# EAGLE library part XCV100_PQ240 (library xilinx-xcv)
xcv100_pq240_1532 edit this description Auto generated by make-symbol-device-package-bsdl.ulp Rev. 26 Source: xcv100_pq240_1532.bsd
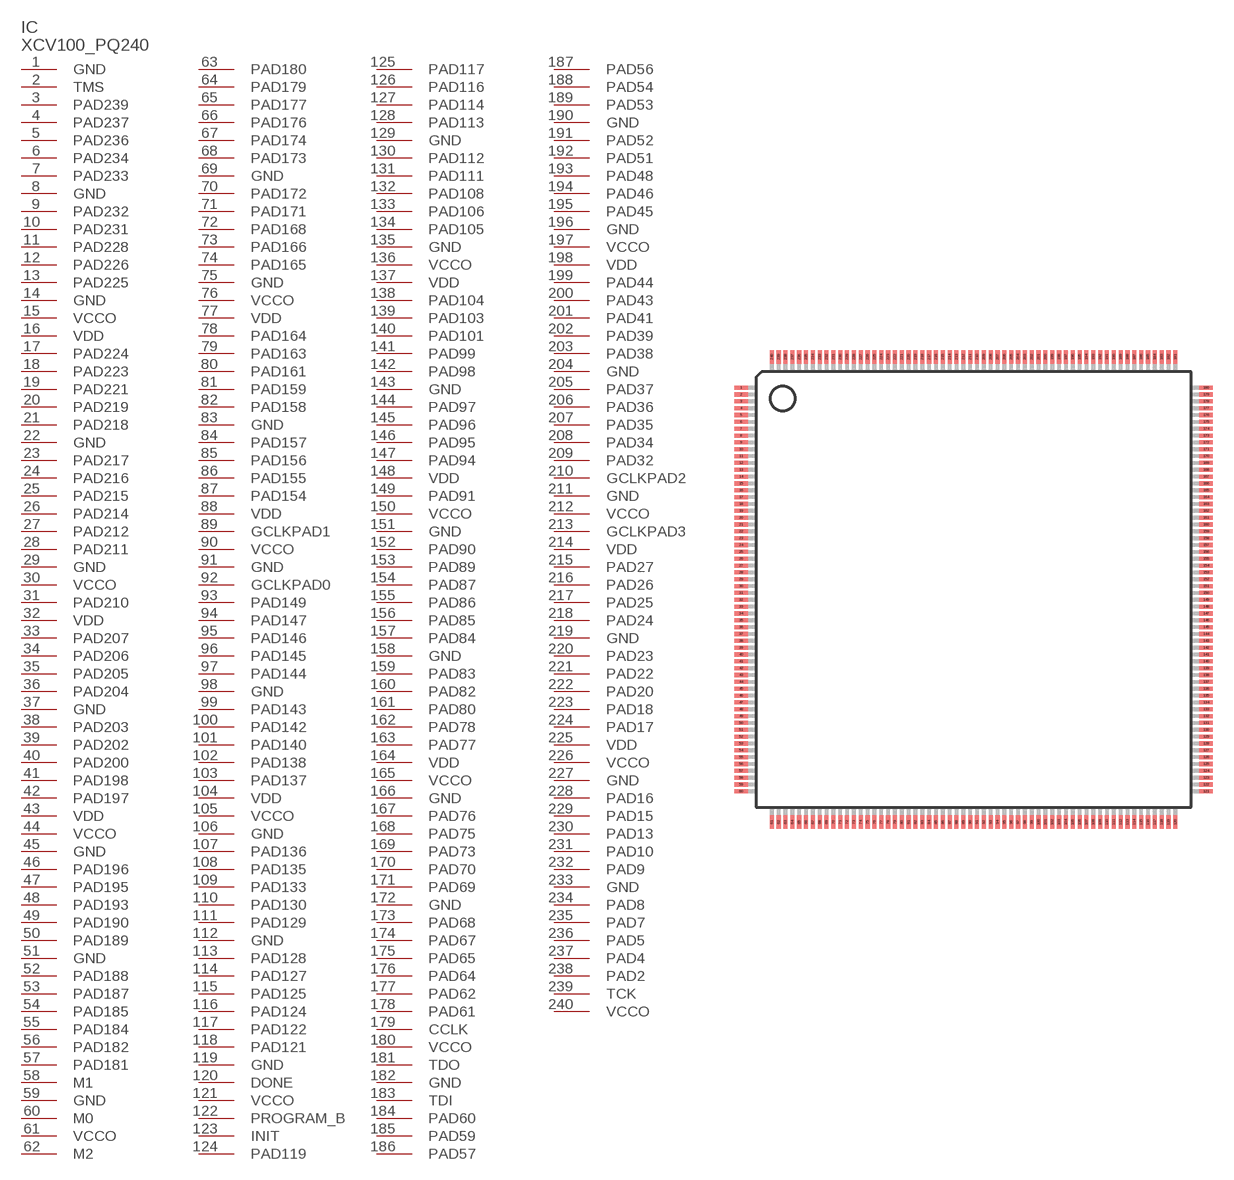
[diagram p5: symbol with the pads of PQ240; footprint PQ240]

Designator prefix IC

## XCV100_PQ240 (OC_FARNELL: unknown; OC_NEWARK: unknown)  [PQ240]
1  GND  pwr
2  TMS  in
3  PAD239
4  PAD237
5  PAD236
6  PAD234
7  PAD233
8  GND  pwr
9  PAD232
10  PAD231
11  PAD228
12  PAD226
13  PAD225
14  GND  pwr
15  VCCO  pwr
16  VDD  pwr
17  PAD224
18  PAD223
19  PAD221
20  PAD219
21  PAD218
22  GND  pwr
23  PAD217
24  PAD216
25  PAD215
26  PAD214
27  PAD212
28  PAD211
29  GND  pwr
30  VCCO  pwr
31  PAD210
32  VDD  pwr
33  PAD207
34  PAD206
35  PAD205
36  PAD204
37  GND  pwr
38  PAD203
39  PAD202
40  PAD200
41  PAD198
42  PAD197
43  VDD  pwr
44  VCCO  pwr
45  GND  pwr
46  PAD196
47  PAD195
48  PAD193
49  PAD190
50  PAD189
51  GND  pwr
52  PAD188
53  PAD187
54  PAD185
55  PAD184
56  PAD182
57  PAD181
58  M1  in
59  GND  pwr
60  M0  in
61  VCCO  pwr
62  M2  in
63  PAD180
64  PAD179
65  PAD177
66  PAD176
67  PAD174
68  PAD173
69  GND  pwr
70  PAD172
71  PAD171
72  PAD168
73  PAD166
74  PAD165
75  GND  pwr
76  VCCO  pwr
77  VDD  pwr
78  PAD164
79  PAD163
80  PAD161
81  PAD159
82  PAD158
83  GND  pwr
84  PAD157
85  PAD156
86  PAD155
87  PAD154
88  VDD  pwr
89  GCLKPAD1  in
90  VCCO  pwr
91  GND  pwr
92  GCLKPAD0  in
93  PAD149
94  PAD147
95  PAD146
96  PAD145
97  PAD144
98  GND  pwr
99  PAD143
100  PAD142
101  PAD140
102  PAD138
103  PAD137
104  VDD  pwr
105  VCCO  pwr
106  GND  pwr
107  PAD136
108  PAD135
109  PAD133
110  PAD130
111  PAD129
112  GND  pwr
113  PAD128
114  PAD127
115  PAD125
116  PAD124
117  PAD122
118  PAD121
119  GND  pwr
120  DONE
121  VCCO  pwr
122  PROGRAM_B  in
123  INIT
124  PAD119
125  PAD117
126  PAD116
127  PAD114
128  PAD113
129  GND  pwr
130  PAD112
131  PAD111
132  PAD108
133  PAD106
134  PAD105
135  GND  pwr
136  VCCO  pwr
137  VDD  pwr
138  PAD104
139  PAD103
140  PAD101
141  PAD99
142  PAD98
143  GND  pwr
144  PAD97
145  PAD96
146  PAD95
147  PAD94
148  VDD  pwr
149  PAD91
150  VCCO  pwr
151  GND  pwr
152  PAD90
153  PAD89
154  PAD87
155  PAD86
156  PAD85
157  PAD84
158  GND  pwr
159  PAD83
160  PAD82
161  PAD80
162  PAD78
163  PAD77
164  VDD  pwr
165  VCCO  pwr
166  GND  pwr
167  PAD76
168  PAD75
169  PAD73
170  PAD70
171  PAD69
172  GND  pwr
173  PAD68
174  PAD67
175  PAD65
176  PAD64
177  PAD62
178  PAD61
179  CCLK
180  VCCO  pwr
181  TDO  out
182  GND  pwr
183  TDI  in
184  PAD60
185  PAD59
186  PAD57
187  PAD56
188  PAD54
189  PAD53
190  GND  pwr
191  PAD52
192  PAD51
193  PAD48
194  PAD46
195  PAD45
196  GND  pwr
197  VCCO  pwr
198  VDD  pwr
199  PAD44
200  PAD43
201  PAD41
202  PAD39
203  PAD38
204  GND  pwr
205  PAD37
206  PAD36
207  PAD35
208  PAD34
209  PAD32
210  GCLKPAD2  in
211  GND  pwr
212  VCCO  pwr
213  GCLKPAD3  in
214  VDD  pwr
215  PAD27
216  PAD26
217  PAD25
218  PAD24
219  GND  pwr
220  PAD23
221  PAD22
222  PAD20
223  PAD18
224  PAD17
225  VDD  pwr
226  VCCO  pwr
227  GND  pwr
228  PAD16
229  PAD15
230  PAD13
231  PAD10
232  PAD9
233  GND  pwr
234  PAD8
235  PAD7
236  PAD5
237  PAD4
238  PAD2
239  TCK  in
240  VCCO  pwr

## Footprint PQ240 (pad centres in mm)
PQ240 Auto generated by make-symbol-device-package-bsdl.ulp Rev. 26
smd 1 x 0.3: 1 -17,14.75; 2 -17,14.25; 3 -17,13.75; 4 -17,13.25; 5 -17,12.75; 6 -17,12.25; 7 -17,11.75; 8 -17,11.25; 9 -17,10.75; 10 -17,10.25; 11 -17,9.75; 12 -17,9.25; 13 -17,8.75; 14 -17,8.25; 15 -17,7.75; 16 -17,7.25; 17 -17,6.75; 18 -17,6.25; 19 -17,5.75; 20 -17,5.25; 21 -17,4.75; 22 -17,4.25; 23 -17,3.75; 24 -17,3.25; 25 -17,2.75; 26 -17,2.25; 27 -17,1.75; 28 -17,1.25; 29 -17,0.75; 30 -17,0.25; 31 -17,-0.25; 32 -17,-0.75; 33 -17,-1.25; 34 -17,-1.75; 35 -17,-2.25; 36 -17,-2.75; 37 -17,-3.25; 38 -17,-3.75; 39 -17,-4.25; 40 -17,-4.75; 41 -17,-5.25; 42 -17,-5.75; 43 -17,-6.25; 44 -17,-6.75; 45 -17,-7.25; 46 -17,-7.75; 47 -17,-8.25; 48 -17,-8.75; 49 -17,-9.25; 50 -17,-9.75; 51 -17,-10.25; 52 -17,-10.75; 53 -17,-11.25; 54 -17,-11.75; 55 -17,-12.25; 56 -17,-12.75; 57 -17,-13.25; 58 -17,-13.75; 59 -17,-14.25; 60 -17,-14.75; 121 17,-14.75; 122 17,-14.25; 123 17,-13.75; 124 17,-13.25; 125 17,-12.75; 126 17,-12.25; 127 17,-11.75; 128 17,-11.25; 129 17,-10.75; 130 17,-10.25; 131 17,-9.75; 132 17,-9.25; 133 17,-8.75; 134 17,-8.25; 135 17,-7.75; 136 17,-7.25; 137 17,-6.75; 138 17,-6.25; 139 17,-5.75; 140 17,-5.25; 141 17,-4.75; 142 17,-4.25; 143 17,-3.75; 144 17,-3.25; 145 17,-2.75; 146 17,-2.25; 147 17,-1.75; 148 17,-1.25; 149 17,-0.75; 150 17,-0.25; 151 17,0.25; 152 17,0.75; 153 17,1.25; 154 17,1.75; 155 17,2.25; 156 17,2.75; 157 17,3.25; 158 17,3.75; 159 17,4.25; 160 17,4.75; 161 17,5.25; 162 17,5.75; 163 17,6.25; 164 17,6.75; 165 17,7.25; 166 17,7.75; 167 17,8.25; 168 17,8.75; 169 17,9.25; 170 17,9.75; 171 17,10.25; 172 17,10.75; 173 17,11.25; 174 17,11.75; 175 17,12.25; 176 17,12.75; 177 17,13.25; 178 17,13.75; 179 17,14.25; 180 17,14.75
smd 0.3 x 1: 61 -14.75,-17; 62 -14.25,-17; 63 -13.75,-17; 64 -13.25,-17; 65 -12.75,-17; 66 -12.25,-17; 67 -11.75,-17; 68 -11.25,-17; 69 -10.75,-17; 70 -10.25,-17; 71 -9.75,-17; 72 -9.25,-17; 73 -8.75,-17; 74 -8.25,-17; 75 -7.75,-17; 76 -7.25,-17; 77 -6.75,-17; 78 -6.25,-17; 79 -5.75,-17; 80 -5.25,-17; 81 -4.75,-17; 82 -4.25,-17; 83 -3.75,-17; 84 -3.25,-17; 85 -2.75,-17; 86 -2.25,-17; 87 -1.75,-17; 88 -1.25,-17; 89 -0.75,-17; 90 -0.25,-17; 91 0.25,-17; 92 0.75,-17; 93 1.25,-17; 94 1.75,-17; 95 2.25,-17; 96 2.75,-17; 97 3.25,-17; 98 3.75,-17; 99 4.25,-17; 100 4.75,-17; 101 5.25,-17; 102 5.75,-17; 103 6.25,-17; 104 6.75,-17; 105 7.25,-17; 106 7.75,-17; 107 8.25,-17; 108 8.75,-17; 109 9.25,-17; 110 9.75,-17; 111 10.25,-17; 112 10.75,-17; 113 11.25,-17; 114 11.75,-17; 115 12.25,-17; 116 12.75,-17; 117 13.25,-17; 118 13.75,-17; 119 14.25,-17; 120 14.75,-17; 181 14.75,17; 182 14.25,17; 183 13.75,17; 184 13.25,17; 185 12.75,17; 186 12.25,17; 187 11.75,17; 188 11.25,17; 189 10.75,17; 190 10.25,17; 191 9.75,17; 192 9.25,17; 193 8.75,17; 194 8.25,17; 195 7.75,17; 196 7.25,17; 197 6.75,17; 198 6.25,17; 199 5.75,17; 200 5.25,17; 201 4.75,17; 202 4.25,17; 203 3.75,17; 204 3.25,17; 205 2.75,17; 206 2.25,17; 207 1.75,17; 208 1.25,17; 209 0.75,17; 210 0.25,17; 211 -0.25,17; 212 -0.75,17; 213 -1.25,17; 214 -1.75,17; 215 -2.25,17; 216 -2.75,17; 217 -3.25,17; 218 -3.75,17; 219 -4.25,17; 220 -4.75,17; 221 -5.25,17; 222 -5.75,17; 223 -6.25,17; 224 -6.75,17; 225 -7.25,17; 226 -7.75,17; 227 -8.25,17; 228 -8.75,17; 229 -9.25,17; 230 -9.75,17; 231 -10.25,17; 232 -10.75,17; 233 -11.25,17; 234 -11.75,17; 235 -12.25,17; 236 -12.75,17; 237 -13.25,17; 238 -13.75,17; 239 -14.25,17; 240 -14.75,17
